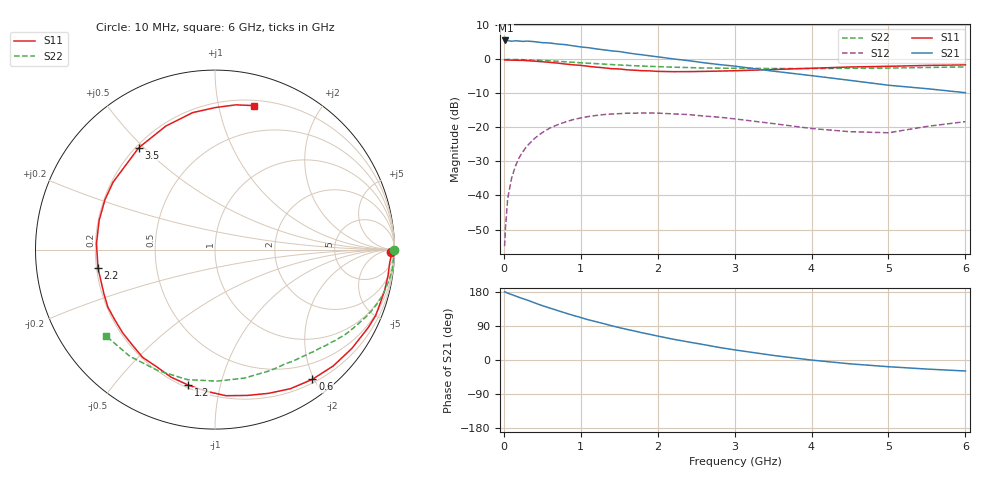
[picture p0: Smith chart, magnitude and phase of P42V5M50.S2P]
! SIEMENS Small Signal Semiconductors
! BFP182
! Si NPN RF Bipolar Junction Transistor in SOT143
! VCE = 2.5 V  IC = 0.5 mA
! Common Emitter S-Parameters:  March  1996
# GHz  S  MA  R  50
!  f  S11  S21  S12  S22
! GHz  MAG  ANG  MAG  ANG  MAG  ANG  MAG  ANG
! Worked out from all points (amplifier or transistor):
!   36 points, 10 MHz to 6 GHz, reference 50 ohm
!   highest |S21| = 5.6 dB at 20 MHz (marker M1)
!   |S21| within 3 dB of that: start of sweep to 1.381 GHz
!   unconditionally stable (mu >= 1): 2.949 GHz to end of sweep
!   at 250 MHz: K = 0.09, MSG = 16.2 dB, |S12| = -27.1 dB
!   at 1.4 GHz: K = 0.49, MSG = 9.3 dB, |S12| = -16.0 dB
!   at 6 GHz: K = 1.20, MAG = 1.6 dB, |S12| = -18.3 dB
!   S11 on the Smith chart (normalised r, x): 10 MHz: 63, -59; 600 MHz: 0.25, -1.98; 1.2 GHz: 0.22, -0.80; 2.2 GHz: 0.21, -0.08; 3.5 GHz: 0.21, +0.48; 6 GHz: 0.25, +1.28
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0.01  0.9832 -0.9  1.855 179.7  0.0018 82.7  0.9993 -0.2
0.02  0.9826 -1.9  1.897 179.3  0.0032 84.6  0.993 -0.6
0.05  0.976 -4.4  1.887 176.4  0.009 89.3  0.9988 -1.6
0.1  0.9747 -8.8  1.849 172.8  0.0178 83.3  0.9954 -3.2
0.15  0.9721 -13.7  1.876 169.1  0.0269 80.8  0.9951 -4.9
0.2  0.9676 -18.2  1.86 165.2  0.0362 78.1  0.9936 -6.5
0.3  0.9582 -26.9  1.857 158.5  0.0531 72.3  0.9851 -9.7
0.4  0.9407 -35.8  1.82 150.7  0.0691 66.9  0.9758 -12.8
0.6  0.9038 -53.1  1.74 137.0  0.0982 55.6  0.9512 -18.6
0.8  0.8549 -69.5  1.648 124.0  0.1203 45.7  0.9215 -23.9
1.1  0.7904 -93.7  1.484 106.1  0.1447 32.2  0.8784 -30.9
1.2  0.7692 -101.2  1.427 101.0  0.1501 27.8  0.8659 -33.2
1.6  0.7033 -130.9  1.251 80.7  0.162 14.1  0.8174 -40.7
1.9  0.6774 -151.8  1.127 67.6  0.1627 5.3  0.7894 -46.1
2.2  0.6601 -171.0  1.017 54.9  0.158 -2.0  0.7683 -51.3
2.8  0.6731 155.7  0.839 33.1  0.1415 -13.3  0.7434 -62.3
3.5  0.709 126.8  0.672 12.1  0.114 -19.1  0.7345 -77.1
4  0.7407 111.7  0.577 -0.2  0.0964 -16.1  0.7329 -89.2
4.5  0.7732 99.3  0.492 -10.1  0.0865 -8.8  0.7406 -102.0
5  0.7913 89.9  0.417 -17.7  0.0835 6.3  0.7454 -115.2
5.5  0.8149 81.8  0.371 -23.9  0.1035 13.5  0.7607 -128.6
6  0.8315 74.7  0.324 -29.0  0.1216 15.0  0.7748 -141.6
